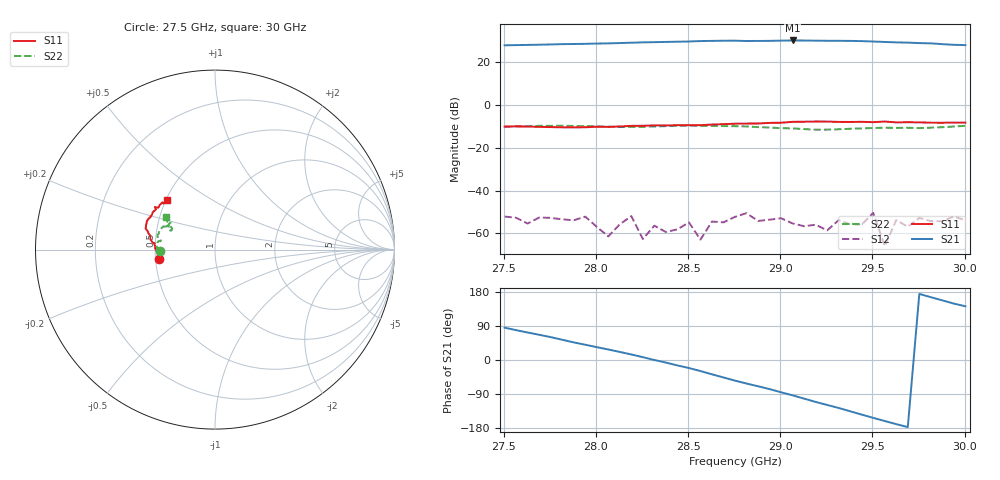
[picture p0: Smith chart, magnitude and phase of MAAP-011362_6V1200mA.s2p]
!Agilent Technologies,E8364C,MY48140145,A.09.42.15
!Agilent E8364C: A.09.42.15
!Date: Friday, June 30, 2023 12:10:23
!Correction: S11(Full 2 Port(1,2))
!S21(Full 2 Port(1,2))
!S12(Full 2 Port(1,2))
!S22(Full 2 Port(1,2))
!S2P File: Measurements: S11, S21, S12, S22:
# Hz S  dB  R 50
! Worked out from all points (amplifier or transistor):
!   41 points, 27.5 GHz to 30 GHz, reference 50 ohm
!   highest |S21| = 30.1 dB at 29.07 GHz (marker M1)
!   |S21| within 3 dB of that: start of sweep to end of sweep
!   unconditionally stable (mu >= 1): start of sweep to end of sweep
!   at 27.88 GHz: K = 7.56, MAG = 29.4 dB, |S12| = -53.8 dB
!   at 28.75 GHz: K = 5.11, MAG = 31.1 dB, |S12| = -52.2 dB
!   at 30 GHz: K = 7.42, MAG = 29.2 dB, |S12| = -53.9 dB
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2.75045e10  -10.08 -170.9  27.87 85.4  -52.09 -58.8  -10.21 -178.1
2.775445e10  -10.32 -175.5  28.27 60.4  -52.70 -88.6  -9.75 176.5
2.794191e10  -10.40 -176.1  28.55 40.3  -52.13 -110.9  -9.88 172.1
2.806689e10  -10.23 -177.1  28.77 27.8  -61.37 -99.6  -10.15 171.2
2.819186e10  -9.75 -177.9  29.08 14.6  -51.89 -33.1  -10.25 171.3
2.825435e10  -9.72 -179.8  29.24 7.5  -62.57 -86.9  -10.23 171.3
2.837932e10  -9.55 177.0  29.44 -6.8  -59.31 -97.0  -9.87 169.4
2.856679e10  -9.43 173.9  29.85 -29.1  -62.85 -122.0  -9.73 164.5
2.869176e10  -8.94 172.2  30.01 -46.1  -54.80 -102.8  -9.84 159.8
2.875425e10  -8.74 170.6  30.03 -54.5  -52.22 -99.2  -9.90 157.8
2.894171e10  -8.36 166.4  29.94 -76.8  -53.56 -89.7  -10.51 154.1
2.906669e10  -7.87 163.2  30.13 -93.3  -55.32 -84.0  -10.93 152.7
2.919166e10  -7.73 157.8  30.04 -110.7  -55.90 -135.0  -11.53 154.1
2.931664e10  -7.90 153.2  29.97 -126.6  -53.77 -146.5  -11.35 156.9
2.944161e10  -7.86 149.0  29.83 -144.1  -55.80 -105.9  -10.91 155.6
2.95041e10  -8.01 145.7  29.64 -152.7  -50.40 -93.4  -10.76 153.0
2.956659e10  -7.73 144.8  29.43 -161.0  -65.92 -77.2  -10.58 153.0
2.962908e10  -8.11 143.6  29.23 -169.3  -53.72 -141.7  -10.69 152.1
2.969156e10  -8.05 141.1  29.12 -177.1  -56.86 -124.1  -10.66 151.0
2.981654e10  -8.28 138.3  28.79 165.7  -54.20 -103.5  -10.59 150.1
2.994151e10  -8.23 135.6  28.09 148.8  -52.06 -129.5  -10.06 149.0
3.0004e10  -8.23 134.1  27.97 141.8  -53.86 -172.7  -9.73 146.6
